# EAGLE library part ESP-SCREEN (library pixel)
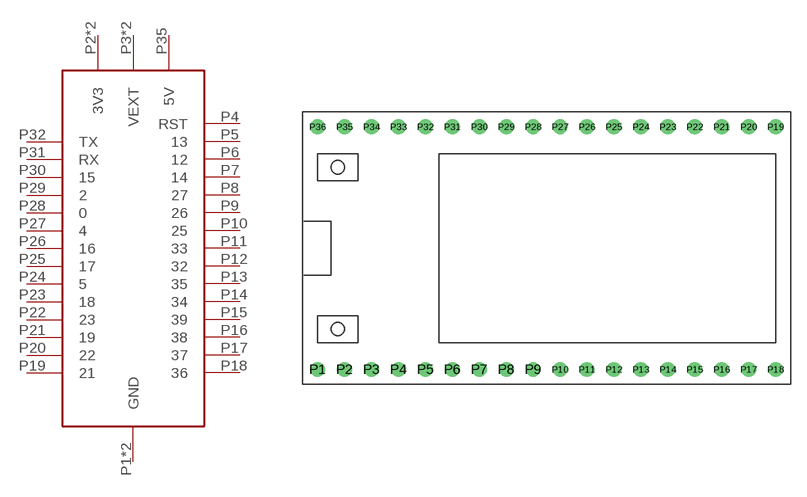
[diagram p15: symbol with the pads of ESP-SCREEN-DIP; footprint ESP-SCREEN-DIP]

Designator prefix -

## ESP-SCREEN  [ESP-SCREEN-DIP]
P1  GND
P2  3V3
P3  VEXT
P4  RST
P5  13
P6  12
P7  14
P8  27
P9  26
P10  25
P11  33
P12  32
P13  35
P14  34
P15  39
P16  38
P17  37
P18  36
P19  21
P20  22
P21  19
P22  23
P23  18
P24  5
P25  17
P26  16
P27  4
P28  0
P29  2
P30  15
P31  RX
P32  TX
P33  VEXT
P34  3V3
P35  5V
P36  GND

## Footprint ESP-SCREEN-DIP (pad centres in mm)
drill 0.9: P1 -21.59,-11.43; P2 -19.05,-11.43; P3 -16.51,-11.43; P4 -13.97,-11.43; P5 -11.43,-11.43; P6 -8.89,-11.43; P7 -6.35,-11.43; P8 -3.81,-11.43; P9 -1.27,-11.43; P10 1.27,-11.43; P11 3.81,-11.43; P12 6.35,-11.43; P13 8.89,-11.43; P14 11.43,-11.43; P15 13.97,-11.43; P16 16.51,-11.43; P17 19.05,-11.43; P18 21.59,-11.43; P19 21.59,11.43; P20 19.05,11.43; P21 16.51,11.43; P22 13.97,11.43; P23 11.43,11.43; P24 8.89,11.43; P25 6.35,11.43; P26 3.81,11.43; P27 1.27,11.43; P28 -1.27,11.43; P29 -3.81,11.43; P30 -6.35,11.43; P31 -8.89,11.43; P32 -11.43,11.43; P33 -13.97,11.43; P34 -16.51,11.43; P35 -19.05,11.43; P36 -21.59,11.43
